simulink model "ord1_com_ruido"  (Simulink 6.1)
settings: Solver=ode45  StartTime=0.0  StopTime=Tfinal  RelTol=1e-6
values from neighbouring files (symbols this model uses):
  Tr = 0.01    [aquisicao_dados.m]    (also in metodo_conv_cov05.m)
  Ts = 0.1    [aquisicao_dados.m]    (also in metodo_conv_cov05.m = 0.2)
undefined symbols (not defined in the file or in its folder): sigbuilder_block
libraries: simulink x1

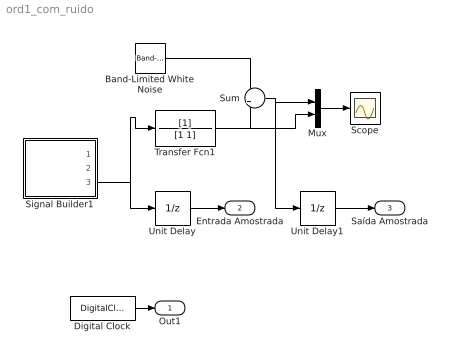
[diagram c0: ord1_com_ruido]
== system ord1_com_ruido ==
  Band-Limited White Noise : simulink/Sources/Band-Limited White Noise  Cov=pr  Ts=Tr  seed=[23341]
  Digital Clock : DigitalClock  SampleTime=Ts
  Mux : Mux  Inputs=2
  Scope : Scope
  Signal Builder1 : Subsystem  Tag=STV Subsys  LoadFcn=sigbuilder_block('load',[18.75 87.75 519.75 399.75 ]);  StartFcn=sigbuilder_block('start');  StopFcn=sigbuilder_block('stop');  ClipboardFcn=sigbuilder_block('clipboard');
  Sum : Sum
  Transfer Fcn1 : TransferFcn  Denominator=[1 1]
  Unit Delay : UnitDelay  SampleTime=Ts
  Unit Delay1 : UnitDelay  SampleTime=Ts
  Out1 : Outport
  Entrada Amostrada : Outport  Port=2
  Saída Amostrada : Outport  Port=3
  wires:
  Band-Limited White Noise/1 -> Sum/1
  Transfer Fcn1/1 -> Sum/2, Mux/2
  Sum/1 -> Mux/1, Unit Delay1/1
  Unit Delay/1 -> Entrada Amostrada/1
  Unit Delay1/1 -> Saída Amostrada/1
  Mux/1 -> Scope/1
  Digital Clock/1 -> Out1/1
  Signal Builder1/3(Signal 4) -> Transfer Fcn1/1, Unit Delay/1

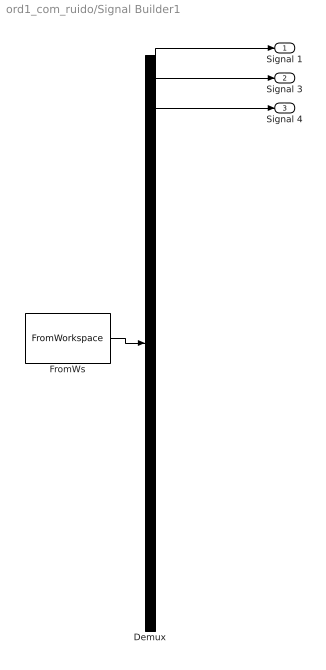
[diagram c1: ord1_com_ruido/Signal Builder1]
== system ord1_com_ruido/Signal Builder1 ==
  Demux : Demux  Tag=STV Demux  Outputs=3
  FromWs : FromWorkspace  Tag=STV FromWs  VariableName=tuvar  SampleTime=0  SigBuilderData=DataTag0  VnvData=DataTag1
  Signal 1 : Outport  Tag=STV Outport
  Signal 3 : Outport  Tag=STV Outport  Port=2
  Signal 4 : Outport  Tag=STV Outport  Port=3
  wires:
  Demux/1 -> Signal 1/1
  FromWs/1 -> Demux/1
  Demux/2 -> Signal 3/1
  Demux/3 -> Signal 4/1
